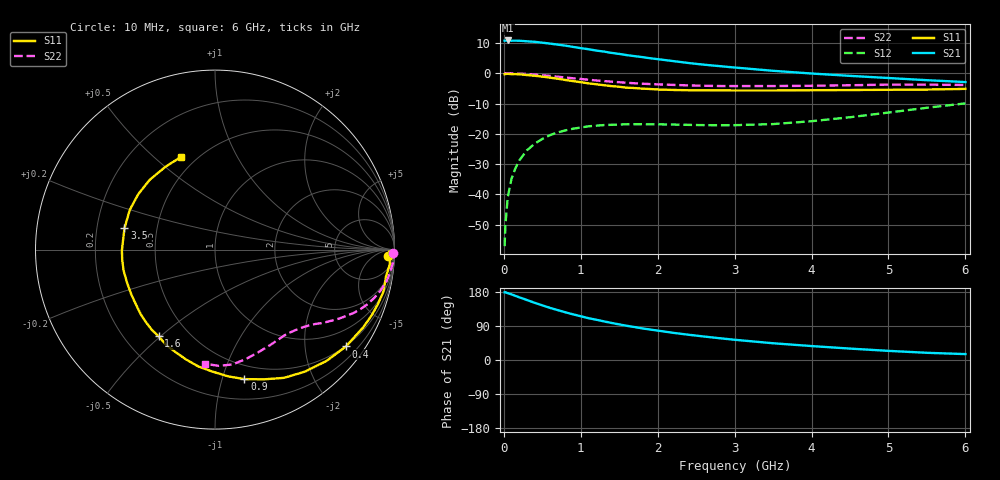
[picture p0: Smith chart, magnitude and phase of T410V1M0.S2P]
! Infineon Technologies  Discrete & RF Semiconductors
! BFR182T
! Si NPN RF Bipolar Junction Transistor in SC75
! VCE = 10 V  IC = 1 mA
! Common Emitter S-Parameters:  October  1999
# GHz  S  MA  R  50
!  f  S11  S21  S12  S22
! GHz  MAG  ANG  MAG  ANG  MAG  ANG  MAG  ANG
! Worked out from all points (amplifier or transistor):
!   36 points, 10 MHz to 6 GHz, reference 50 ohm
!   highest |S21| = 10.8 dB at 50 MHz (marker M1)
!   |S21| within 3 dB of that: start of sweep to 1.125 GHz
!   unconditionally stable (mu >= 1): 2.464 GHz to 4.65 GHz
!   at 250 MHz: K = 0.09, MSG = 18.9 dB, |S12| = -27.1 dB
!   at 1.4 GHz: K = 0.57, MSG = 11.9 dB, |S12| = -17.0 dB
!   at 6 GHz: K = 0.84, MSG = 3.5 dB, |S12| = -10.0 dB
!   S11 on the Smith chart (normalised r, x): 10 MHz: 29, -27; 400 MHz: 0.48, -2.96; 900 MHz: 0.37, -1.18; 1.6 GHz: 0.34, -0.49; 3.5 GHz: 0.32, +0.10; 6 GHz: 0.41, +0.62
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0.01  0.9642 -2.0  3.447 178.6  0.0014 87.0  0.9915 -1.1
0.02  0.9714 -0.5  3.437 178.9  0.0031 96.9  0.9992 -0.7
0.05  0.9776 -4.8  3.47 176.4  0.0089 90.1  0.9958 -1.8
0.1  0.9646 -8.8  3.437 173.2  0.0182 86.0  0.9964 -3.6
0.2  0.9572 -18.5  3.43 165.5  0.0362 80.0  0.9845 -7.2
0.3  0.9331 -27.5  3.359 158.3  0.0533 74.0  0.9704 -10.7
0.4  0.9076 -36.5  3.296 151.0  0.0686 68.5  0.9498 -14.0
0.5  0.8781 -44.9  3.189 144.3  0.0822 63.5  0.9268 -16.9
0.6  0.8446 -53.6  3.08 137.6  0.0951 59.3  0.9026 -19.7
0.8  0.773 -69.2  2.849 125.9  0.1139 51.4  0.85 -24.5
0.9  0.74 -77.2  2.716 120.4  0.1215 48.4  0.8246 -26.4
1.1  0.6795 -91.3  2.488 110.4  0.1331 42.7  0.7803 -29.9
1.3  0.6335 -104.6  2.278 102.0  0.1394 38.3  0.7415 -32.9
1.4  0.6126 -110.9  2.163 97.8  0.1408 36.2  0.7252 -34.3
1.6  0.5763 -123.0  1.986 90.2  0.1439 33.7  0.6953 -36.6
1.8  0.557 -134.2  1.846 83.4  0.1443 31.9  0.6711 -39.1
2.2  0.529 -152.1  1.586 71.8  0.1422 31.0  0.6413 -43.5
2.8  0.5202 -173.6  1.31 57.6  0.1386 34.3  0.6147 -51.1
3.5  0.5184 166.8  1.096 44.2  0.1447 43.9  0.6143 -60.0
4.5  0.5274 144.2  0.904 30.1  0.1878 56.7  0.633 -74.0
5.5  0.5374 121.2  0.767 19.0  0.2692 59.8  0.648 -88.1
6  0.5509 109.9  0.714 15.6  0.3179 57.8  0.6389 -94.8
